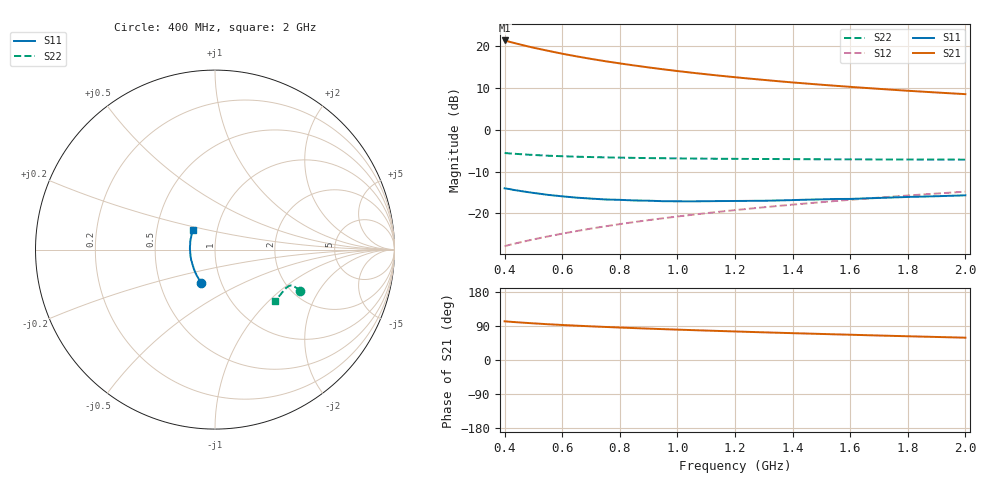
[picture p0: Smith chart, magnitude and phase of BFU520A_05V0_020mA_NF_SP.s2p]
! Filename:  P:\Prog\Test\Noise\ATS_data\Testdata_Net\06 Compressed Noise after Statistics\BFU520A_APG2013_30_A05_05p0V_020mA_NF_CM01_D.sf
! Date/Time: Wed 24/Apr/2013 20:06:18
! BFU520A_APG2013_30_A05_05p0V_1to20mA_NF_CM01_Bias8_R.sf
! Noise Parameter Data File
! BFU520A_APG2013_30_A05_05p0V_1to20mA_NF_CM01
! Date/time: Thu Apr 11 01:07:08 2013
! VAR V_out= 5.001000
! VAR I_out= 19.995000
! VAR V_in= 0.849500
! VAR I_in= 0.227950
! Device data file deembeded for feedlines and parallel
! Original file: \06 Compressed Noise after Statistics\BFU520A_APG2013_30_A05_05p0V_020mA_NF_CM01_R.sf
! Feed-files: PR017V01_150413_Feed1.s2p, PR017V01_150413_Feed2.s2p
! Parallel-file: PR017V01_150413_Par.s2p
# MHz S MA R 50
!  Freq-MHz  S11-mag  S11-arg  S21-mag  S21-arg  S12-mag  S12-arg  S22-mag  S22-arg
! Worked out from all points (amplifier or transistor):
!   37 points, 400 MHz to 2 GHz, reference 50 ohm
!   highest |S21| = 21.4 dB at 400 MHz (marker M1)
!   |S21| within 3 dB of that: start of sweep to 587.5 MHz
!   unconditionally stable (mu >= 1): 855.3 MHz to 1.716 GHz
!   at 500 MHz: K = 0.94, MSG = 23.0 dB, |S12| = -26.3 dB
!   at 1.1 GHz: K = 1.01, MAG = 16.1 dB, |S12| = -20.0 dB
!   at 2 GHz: K = 0.99, MSG = 11.7 dB, |S12| = -14.8 dB
!   lowest NFmin = 1.11 dB at 420 MHz
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400  0.1991 -112.5  11.8 102.1  0.04029 73.5  0.5275 -25.6
420  0.1942 -115.4  11.3 100.9  0.04199 73.7  0.5207 -25.5
440  0.1885 -118.2  10.85 99.8  0.04362 73.9  0.5149 -25.4
460  0.1838 -120.6  10.42 98.7  0.04528 74.1  0.5097 -25.3
480  0.1795 -123.2  10.03 97.7  0.04691 74.3  0.5043 -25.2
500  0.1755 -125.9  9.667 96.8  0.0486 74.4  0.5002 -25.2
550  0.1662 -132.0  8.882 94.4  0.0527 74.8  0.4897 -25.0
600  0.1596 -137.4  8.185 92.4  0.05695 75.1  0.4829 -24.9
650  0.1538 -142.5  7.603 90.6  0.06117 75.3  0.4766 -25.1
700  0.1499 -147.3  7.096 88.8  0.06546 75.6  0.4718 -25.1
750  0.1463 -152.0  6.651 87.2  0.06975 75.7  0.4677 -25.3
800  0.1448 -156.4  6.262 85.7  0.07404 75.8  0.4644 -25.6
850  0.1424 -160.9  5.917 84.2  0.07837 75.8  0.4611 -25.9
950  0.1395 -168.8  5.324 81.4  0.08704 75.8  0.4566 -26.7
1050  0.1388 -175.7  4.846 78.9  0.09575 75.7  0.4528 -27.6
1150  0.14 177.5  4.449 76.5  0.1046 75.5  0.4498 -28.6
1200  0.1403 174.7  4.277 75.3  0.109 75.3  0.449 -29.2
1350  0.1424 166.1  3.83 71.9  0.1224 74.8  0.4466 -31.0
1500  0.1467 158.4  3.476 68.7  0.1358 74.2  0.4435 -33.0
1650  0.1507 151.8  3.187 65.6  0.1495 73.4  0.4424 -35.2
1750  0.1547 147.7  3.019 63.6  0.1585 72.9  0.4411 -36.6
2000  0.164 138.9  2.681 58.9  0.1815 71.5  0.4394 -40.6
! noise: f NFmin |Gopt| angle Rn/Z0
400  1.19  0.2148  -163.4  0.0992
460  1.145  0.2295  -161.2  0.0979
600  1.3  0.2098  -156.4  0.1098
800  1.184  0.2718  -153.9  0.0908
1000  1.248  0.2716  -147.2  0.0974
1200  1.306  0.285  -141.3  0.1037
1400  1.341  0.2997  -134.9  0.1135
1600  1.342  0.3228  -129.7  0.1197
1800  1.394  0.3551  -128  0.1108
2000  1.362  0.3567  -119.9  0.1423
